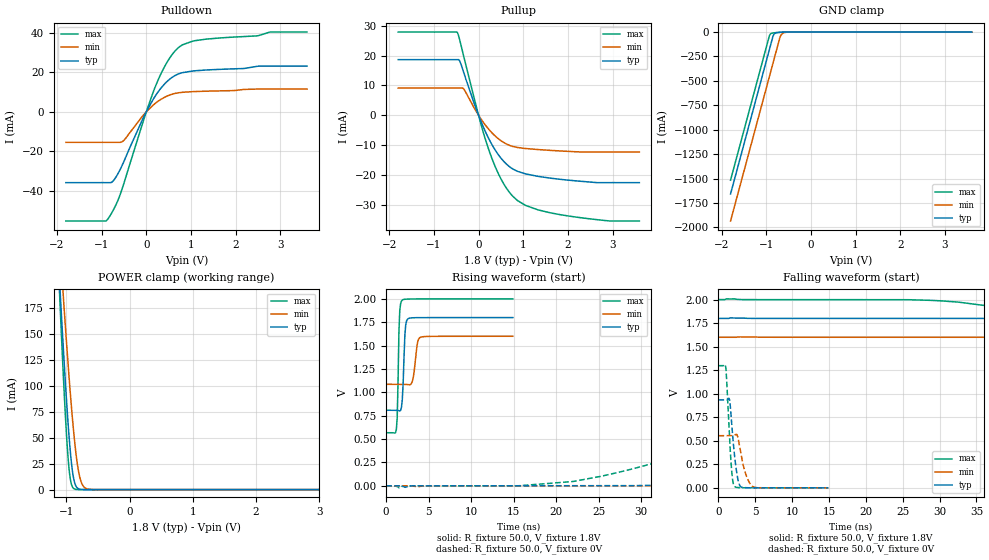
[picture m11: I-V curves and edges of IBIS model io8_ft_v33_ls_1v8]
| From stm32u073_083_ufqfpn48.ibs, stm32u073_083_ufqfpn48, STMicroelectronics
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[Model]   io8_ft_v33_ls_1v8
Model_type I/O
Polarity   Non-Inverting
Enable   Active-Low
| CAP_THRESHOLD on pad IOFT is "UDTCAPC" :
| Rising=30.0% of vddiom   Falling=70.0% of vddiom
| C_comp min and max val. don't necessarily correlate with the min and max pvt
| but are the smallest and greatest pad capacitance found.
| var   typ   min   max
C_comp   2.10723pF  2.10452pF  2.16862pF
|C_comp_pullup   1.19917pF  1.17985pF  1.18495pF
|C_comp_pulldown   908.05315fF  924.66568fF  983.67002fF
Vinl = 480.0mV
Vinh = 1.4V
Vmeas = 900.0mV   | Reference voltage for timing measurements
Cref  = 50.0pF   | Timing specification test load capacitance value
Rref  = 100.0MOhm   | Timing specification test load resistance value
Vref  = 900.0mV   | Timing specification test load voltage
[Model Spec]
| TIME_THRESHOLD on pin ZIV33M is "CMOS" :
| Rising=50.0% of vddiom   Falling=50.0% of vddiom
Vinl 728.70000mV 655.70000mV 817.70000mV
Vinh 1.06430V 949.30000mV 1.16330V
| variable   typ   min   max
[Temperature Range] 25.0 140.0 -40.0
| variable   typ   min   max
[Voltage Range] 1.8V 1.6V 2.0V
| variable   typ   min   max
[POWER Clamp Reference] 1.8V 1.6V 2.0V
| variable   typ   min   max
[GND Clamp Reference] 0V 0V 0V
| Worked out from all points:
|   slope of the pulldown table from 0 to 0.27 V, typ, clamps not added: 26.3 ohm
|   slope of the pullup table from 0 to 0.27 V, typ, clamps not added: 30 ohm
|   GND clamp passes 1 mA (typ) near -0.61 V on its own axis
|   POWER clamp passes 1 mA (typ) near -0.81 V on its own axis
|   rising waveform, R_fixture 50.0, V_fixture 1.8V: 20-80 % time 251ps typ, 393ps min, 199ps max; typ from 0.809 V to 1.8 V
|   falling waveform, R_fixture 50.0, V_fixture 1.8V: 20-80 % time 67ns typ, 120ns min, 35.2ns max; typ from 1.8 V to 0.809 V
|   rising waveform, R_fixture 50.0, V_fixture 0V: 20-80 % time 65.2ns typ, 121ns min, 35.8ns max; typ from 0 V to 0.935 V
|   falling waveform, R_fixture 50.0, V_fixture 0V: 20-80 % time 695ps typ, 1.01ns min, 535ps max; typ from 0.935 V to 0 V
[POWER Clamp]
-1.8V     1.053A     943.1mA    1.262A
-1.11V    202.2mA    242.3mA    190.9mA
-1.09V    180mA      223.6mA    163.4mA
-1.05V    136.9mA    187mA      110.9mA
-980mV    68.91mA    126.1mA    35.23mA
-940mV    37.57mA    94.11mA    10.65mA
-880mV    8.969mA    52.17mA    807.4uA
-830mV    1.697mA    25.82mA    75.79uA
-790mV    394.2uA    12.22mA    11.25uA
-740mV    61.25uA    3.879mA    1.034uA
-660mV    3.073uA    483.4uA    22.7nA
3.6V      0A         0A         0A
[GND Clamp]
-1.8V     -1.658A    -1.935A    -1.517A
-930mV    -179mA     -456mA     -38.91mA
-900mV    -128mA     -405mA     -17.65mA
-850mV    -44.09mA   -320mA     -9.519mA
-830mV    -24.74mA   -286mA     -8.302mA
-790mV    -9.695mA   -218mA     -6.49mA
-700mV    -2.938mA   -65mA      -3.294mA
-670mV    -2.157mA   -31.85mA   -2.435mA
-640mV    -1.545mA   -16.21mA   -1.699mA
-570mV    -571.9uA   -3.807mA   -536.5uA
-420mV    -14.26uA   -143.3uA   -5.434uA
3.6V      449.1pA    102.3nA    316.4pA
| variable   typ   min   max
[Pullup Reference] 1.8V 1.6V 2.0V
| variable   typ   min   max
[Pulldown Reference] 0V 0V 0V
[Pullup]
-1.8V     18.63mA    9.13mA     27.86mA
-480mV    18.63mA    9.13mA     27.8mA
-420mV    18.05mA    9.13mA     25.03mA
-330mV    14.19mA    8.744mA    19.54mA
40mV      -1.53mA    -918.5uA   -2.253mA
250mV     -8.43mA    -5.045mA   -12.43mA
540mV     -15mA      -8.866mA   -22.31mA
870mV     -18.72mA   -10.75mA   -28.48mA
1.33V     -20.4mA    -11.44mA   -31.6mA
1.9V      -21.5mA    -11.96mA   -33.39mA
2.94V     -22.49mA   -12.26mA   -35.33mA
3.6V      -22.49mA   -12.26mA   -35.33mA
[Pulldown]
-1.8V     -35.76mA   -15.41mA   -55.17mA
-910mV    -35.76mA   -15.41mA   -55.17mA
-830mV    -35.76mA   -15.41mA   -53.18mA
-710mV    -34mA      -15.41mA   -48.42mA
-520mV    -26.05mA   -14.75mA   -37.5mA
-90mV     -4.145mA   -2.306mA   -6.327mA
230mV     8.974mA    4.797mA    14.24mA
490mV     15.87mA    8.222mA    26.01mA
750mV     19.43mA    9.742mA    33.01mA
1.33V     21.16mA    10.45mA    36.75mA
2.78V     23.13mA    11.52mA    40.36mA
3.6V      23.13mA    11.52mA    40.37mA
[Ramp]
dV/dt_r 560.7334mV/65.18145ns 332.39542mV/119.67885ns 778.78019mV/35.81994ns
dV/dt_f 594.84476mV/67.00581ns 308.28383mV/119.27462ns 859.12992mV/35.18084ns
R_load = 50.0
| Removed startup time: 0s 0s 0s  .
| Removed end time: 14.9ns.
[Rising Waveform]
R_fixture   = 50.0
V_fixture   = 1.8V
V_fixture_min = 1.6V
V_fixture_max = 2.0V
0s        808.6mV    1.086V     568.1mV
1.2ns     808.3mV    1.086V     602.7mV
1.3ns     807.6mV    1.086V     729.4mV
1.5ns     803.6mV    1.086V     1.642V
1.6ns     801.5mV    1.086V     1.872V
1.9ns     924.4mV    1.086V     1.988V
2.2ns     1.608V     1.085V     1.996V
2.6ns     1.789V     1.082V     1.998V
4ns       1.799V     1.587V     1.999V
14.9ns    1.8V       1.6V       2V
| Removed startup time: 0s 0s 0s  .
| Removed end time: 999.9ns.
[Falling Waveform]
R_fixture   = 50.0
V_fixture   = 1.8V
V_fixture_min = 1.6V
V_fixture_max = 2.0V
0s        1.8V       1.6V       2V
36.6ns    1.8V       1.6V       1.934V
57.8ns    1.777V     1.6V       1.46V
73.7ns    1.693V     1.598V     1.04V
84.7ns    1.601V     1.594V     831mV
104.9ns   1.391V     1.573V     678.3mV
132.4ns   1.123V     1.519V     613.6mV
188ns     900.3mV    1.345V     578.5mV
315.8ns   817.3mV    1.14V      568.4mV
999.9ns   808.6mV    1.086V     568.1mV
| Removed startup time: 0s 0s 0s  .
| Removed end time: 999.9ns.
[Rising Waveform]
R_fixture   = 50.0
V_fixture   = 0V
V_fixture_min = 0V
V_fixture_max = 0V
0s        -9.652uV   -5.561uV   -9.618uV
22ns      658.3uV    -25.25uV   46.57mV
41.2ns    40.35mV    848.7uV    498.2mV
55.9ns    161.2mV    6.11mV     840.8mV
71ns      322.4mV    21.41mV    1.075V
107.9ns   657.1mV    113.7mV    1.263V
138.6ns   809.8mV    219.9mV    1.289V
174.3ns   888.1mV    331.7mV    1.297V
326.1ns   933.7mV    529.3mV    1.298V
999.9ns   934.6mV    554mV      1.298V
| Removed startup time: 0s 0s 0s  .
| Removed end time: 14.9ns.
[Falling Waveform]
R_fixture   = 50.0
V_fixture   = 0V
V_fixture_min = 0V
V_fixture_max = 0V
0s        934.6mV    554mV      1.298V
1ns       933.9mV    554mV      1.277V
1.5ns     936.5mV    553.7mV    528.7mV
1.7ns     777.7mV    553.5mV    272.9mV
1.9ns     576.1mV    553.8mV    93.82mV
2.2ns     325.8mV    560.3mV    14.4mV
2.9ns     23.13mV    422.8mV    1.748mV
3.6ns     2.107mV    170.3mV    883.3uV
4.6ns     672.7uV    15.53mV    516.3uV
14.9ns    64.68uV    45.44uV    114.2uV
